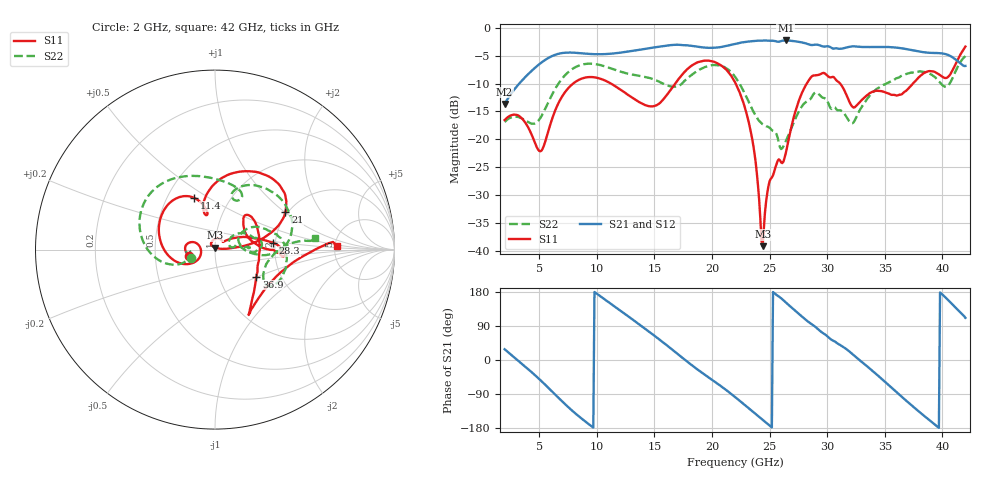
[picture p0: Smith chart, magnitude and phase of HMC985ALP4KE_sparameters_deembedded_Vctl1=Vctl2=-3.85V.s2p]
!s2p File: Measurements: S11, S21, S12, S22
# GHz S dB R 50.0
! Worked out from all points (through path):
!   401 points, 2 GHz to 42 GHz, reference 50 ohm
!   highest |S21| = -2.25 dB at 26.4 GHz (marker M1); lowest = -13.7 dB at 2 GHz (marker M2)
!   lowest |S11| = -39.2 dB at 24.4 GHz (marker M3), VSWR 1.02, Z = 50 + j1.1 ohm
!   |S11| at or under -10 dB: start of sweep to 7.94 GHz; 22.06 GHz to 28.23 GHz (6.165 GHz wide, 24.5 % of centre); 31.13 GHz to 37.44 GHz (6.31 GHz wide, 18.4 % of centre)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
!   |S22| runs from -21.8 to -5.1 dB; largest |S21 - S12| = 0.00066
!   S11 on the Smith chart (normalised r, x): 2 GHz: 0.75, -0.05; 11.4 GHz: 0.68, +0.43; 21 GHz: 1.94, +1.01; 28.3 GHz: 1.95, +0.17; 36.9 GHz: 1.50, -0.49; 42 GHz: 5.23, +0.39
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2  -16.54 -166.3  -13.67 28.5  -13.67 28.5  -16.89 -160.9
3.4  -16.05 168.1  -9.69 -7.6  -9.69 -7.6  -16.16 -178.4
5.1  -22.16 -174.1  -6.36 -52.9  -6.36 -52.9  -16.18 -161.7
6.8  -12.99 -162.3  -4.59 -103.5  -4.59 -103.5  -9.62 -171.4
8.7  -9.09 149.5  -4.55 -155.0  -4.55 -155.0  -6.60 150.5
11.4  -10.19 111.7  -4.59 144.4  -4.59 144.4  -7.38 106.2
13.6  -13.21 102.0  -3.96 95.9  -3.96 95.9  -8.57 75.6
15.4  -13.62 106.3  -3.37 54.9  -3.37 54.9  -9.63 62.9
17.9  -7.31 78.4  -3.13 -5.3  -3.13 -5.3  -9.01 71.2
21  -7.05 28.1  -3.34 -74.0  -3.34 -74.0  -6.93 16.8
22  -9.74 16.8  -2.86 -97.6  -2.86 -97.6  -8.75 -0.1
23.4  -18.94 5.7  -2.39 -132.5  -2.39 -132.4  -14.19 -4.8
24.4  -39.19 87.2  -2.27 -157.7  -2.26 -157.7  -17.29 9.2
25  -27.53 122.1  -2.29 -173.0  -2.29 -173.0  -17.92 12.5
26.4  -22.55 40.5  -2.25 152.2  -2.25 152.2  -20.37 33.8
28.3  -9.74 6.7  -2.87 102.3  -2.87 102.3  -13.10 18.2
28.7  -8.64 0.6  -3.07 93.8  -3.08 93.8  -12.27 15.4
32.4  -14.24 31.1  -3.31 10.2  -3.31 10.2  -16.58 27.0
35.4  -11.83 16.1  -3.43 -67.9  -3.43 -67.9  -9.74 17.9
36.9  -11.21 -33.2  -3.80 -108.4  -3.80 -108.3  -8.23 4.6
39.7  -8.32 -56.6  -4.52 -179.1  -4.52 -179.1  -9.58 -33.9
42  -3.34 1.7  -6.82 111.2  -6.83 111.2  -5.05 6.8
